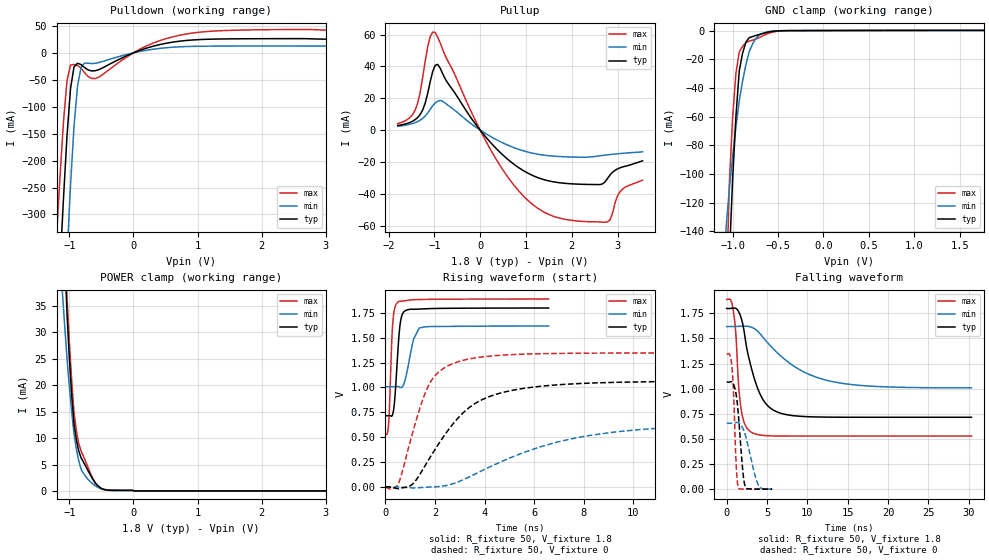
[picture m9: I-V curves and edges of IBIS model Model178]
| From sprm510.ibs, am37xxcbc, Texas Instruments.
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| Model based on original model for DSIPHY_WIO_CORE_GPIOWRAPPER
|   Sub model FBPB_HS00L11_PD1_1P8
[model]   Model178
|[Input Load]   PD
|[Output Drive] SC00LB11
|Voltage   1.8V
|Mode   I/O
Model_type   I/O
Polarity   Non-Inverting
Enable   Active-Low
Vinl =  0.63
Vinh =  1.17
Cref =  15pF
Rref =  100.0000M
Vref =  0V
Vmeas =  0.9
C_comp   1.429432p   1.270657p   1.602015p
[Model Spec]
Vinl   0.63   0.567   0.6615
Vinh   1.17   1.053   1.2285
[Temperature Range]   25   125   -40
[Voltage Range]   1.8   1.62   1.89
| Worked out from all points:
|   slope of the pulldown table from 0 to 0.27 V, typ, clamps not added: 24.3 ohm
|   slope of the pullup table from 0 to 0.27 V, typ, clamps not added: 29.7 ohm
|   GND clamp passes 1 mA (typ) near -0.60 V on its own axis
|   POWER clamp passes 1 mA (typ) near -0.55 V on its own axis
|   rising waveform, R_fixture 50, V_fixture 1.8: 20-80 % time 177ps typ, 312ps min, 125ps max; typ from 0.716 V to 1.8 V
|   rising waveform, R_fixture 50, V_fixture 0: 20-80 % time 2.11ns typ, 4.77ns min, 1.08ns max; typ from 0 V to 1.06 V
|   falling waveform, R_fixture 50, V_fixture 1.8: 20-80 % time 2.08ns typ, 5.9ns min, 724ps max; typ from 1.8 V to 0.716 V
|   falling waveform, R_fixture 50, V_fixture 0: 20-80 % time 643ps typ, 1.17ns min, 383ps max; typ from 1.06 V to 0 V
[POWER_clamp]
-1.8V     362.5mA    191.4mA    412.8mA
-1.109V   56.74mA    37.73mA    60.49mA
-1.073V   44.66mA    31.25mA    47.92mA
-1.036V   33.51mA    25.07mA    36.71mA
-1V       25.05mA    19.75mA    28.19mA
-963.6mV  18.1mA     14.99mA    20.91mA
-927.3mV  12.67mA    10.8mA     14.87mA
-890.9mV  9.735mA    7.937mA    11.45mA
-818.2mV  6.3mA      4.158mA    7.553mA
-563.6mV  1.102mA    739.7uA    992.8uA
18.18mV   0A         0A         0A
3.6V      0A         0A         0A
[Pulldown]
-1.8V     -1.718A    -2.61A     -1.406A
-1.2V     -527.4mA   -844.5mA   -339.9mA
-1.145V   -396mA     -683.1mA   -229.1mA
-1.091V   -269mA     -526.7mA   -127.5mA
-1.036V   -153.6mA   -378.9mA   -51.17mA
-981.8mV  -66.33mA   -245.6mA   -22.67mA
-927.3mV  -26mA      -136.2mA   -21.54mA
-872.7mV  -19.34mA   -61.98mA   -23.69mA
-763.6mV  -27.2mA    -19.05mA   -36.72mA
-545.5mV  -31.39mA   -18.17mA   -45.46mA
872.7mV   23.46mA    11.88mA    35.92mA
3.545V    25.34mA    12.51mA    41.58mA
[Pullup]
-1.8V     2.903mA    2.423mA    4.112mA
-1.418V   6.595mA    4.711mA    12.64mA
-1.255V   12.69mA    7.42mA     33.24mA
-1.091V   30.4mA     13mA       58.69mA
-981.8mV  40.63mA    17.02mA    61.3mA
-818.2mV  35.38mA    18.12mA    50.59mA
272.7mV   -9.18mA    -4.728mA   -14.55mA
1.255V    -29.75mA   -15.09mA   -48.97mA
2.564V    -34.17mA   -16.31mA   -57.57mA
2.782V    -30.25mA   -15.5mA    -57.48mA
3.055V    -23.63mA   -14.68mA   -38.61mA
3.545V    -19.25mA   -13.56mA   -31.41mA
[GND_clamp]
-1.8V     -2.82A     -1.192A    -3.165A
-1.073V   -235.8mA   -138.4mA   -192.1mA
-1.036V   -159.6mA   -110.8mA   -107.6mA
-1V       -103.8mA   -87.86mA   -60.71mA
-963.6mV  -60.04mA   -67.29mA   -29.85mA
-927.3mV  -28.26mA   -49.1mA    -14.96mA
-890.9mV  -15.95mA   -35.5mA    -11.07mA
-854.5mV  -8.194mA   -24.09mA   -8.535mA
-818.2mV  -4.986mA   -14.87mA   -7.361mA
-709.1mV  -2.849mA   -3.094mA   -4.979mA
-563.6mV  -632.2uA   -437.1uA   -1.183mA
1.764V    97.78uA    55.01uA    156.3uA
[Ramp]
dV/dt_f  0.6523168/2.084435n   0.369165/5.947712n   0.8183304/0.7236667n
dV/dt_r  0.6504172/2.122186n   0.3999402/4.817769n   0.8229094/1.082608n
R_load = 50
[Rising Waveform]
R_fixture = 50
V_fixture = 1.8
V_fixture_min = 1.62
V_fixture_max = 1.89
0s        715.6mV    1.007V     530.1mV
126ps     716.3mV    1.007V     633.9mV
252ps     711mV      1.007V     1.457V
306ps     743.8mV    1.007V     1.684V
504ps     1.379V     1.008V     1.858V
585ps     1.624V     1V         1.866V
702ps     1.746V     1.013V     1.869V
1.134ns   1.785V     1.484V     1.881V
1.359ns   1.787V     1.596V     1.883V
6.588ns   1.798V     1.617V     1.888V
[Rising Waveform]
R_fixture = 50
V_fixture = 0
V_fixture_min = 0
V_fixture_max = 0
0s        -243.1uV   72.05uV    -4.557mV
540ps     -17.75mV   494.9uV    43.85mV
1.161ns   45.63mV    -10.54mV   602.4mV
1.863ns   322.4mV    -630.6uV   1.072V
2.502ns   560.8mV    17.23mV    1.215V
3.51ns    821.2mV    116.2mV    1.292V
4.869ns   957.6mV    275.1mV    1.326V
6.75ns    1.022V     438.1mV    1.341V
10.3ns    1.056V     577.1mV    1.346V
31.24ns   1.065V     654.4mV    1.346V
[Falling Waveform]
R_fixture = 50
V_fixture = 1.8
V_fixture_min = 1.62
V_fixture_max = 1.89
0s        1.798V     1.619V     1.888V
891ps     1.803V     1.618V     1.737V
1.179ns   1.797V     1.619V     1.492V
1.548ns   1.757V     1.621V     962.2mV
1.89ns    1.677V     1.622V     748.8mV
3.105ns   1.193V     1.611V     564.3mV
4.842ns   852mV      1.478V     533.1mV
7.065ns   747.8mV    1.301V     528.6mV
13.85ns   716.2mV    1.059V     528.2mV
30.35ns   715.5mV    1.009V     528.2mV
[Falling Waveform]
R_fixture = 50
V_fixture = 0
V_fixture_min = 0
V_fixture_max = 0
0s        1.065V     656mV      1.346V
432ps     1.068V     656mV      1.328V
675ps     1.065V     655.9mV    1.196V
864ps     1.041V     657.2mV    934.5mV
1.188ns   933.5mV    662.7mV    224.3mV
1.431ns   758.9mV    661.3mV    15.53mV
2.034ns   153.2mV    600mV      785.5uV
2.34ns    16.85mV    530.8mV    339uV
3.87ns    409.4uV    50.34mV    40.24uV
5.634ns   126.4uV    1.63mV     8.016uV
